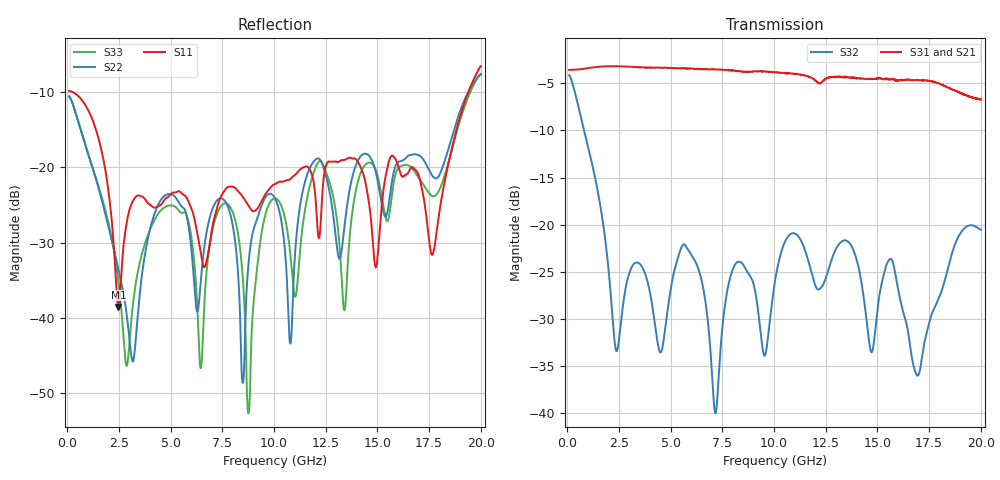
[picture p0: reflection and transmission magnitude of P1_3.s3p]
!The following data was pulled from an Agilent PNA
!This sNp file was generated from the data in the RF Test software
!NOTE:  Smoothing/Math/Corrections applied on any given trace ARE included in the data saved here
# MHz S dB R 50
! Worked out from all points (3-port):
!   6401 points, 100 MHz to 20 GHz, reference 50 ohm
!   strongest paths, dB at 100 MHz, 5.075 GHz, 10.05 GHz, 15.03 GHz, 20 GHz:
!     S31: -3.6, -3.4, -3.8, -4.5, -6.7
!     S21: -3.6, -3.4, -3.9, -4.6, -6.9
!     S32: -4.1, -26.0, -26.0, -28.6, -20.5
!   lowest |S11| = -38.5 dB at 2.485 GHz (marker M1), VSWR 1.02, Z = 49.9 + j1.17 ohm
!   |S11| at or under -10 dB: 236.6 MHz to 19.4 GHz (19.16 GHz wide, 195 % of centre)
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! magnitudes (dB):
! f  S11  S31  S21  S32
! 100 MHz  -9.9  -3.6  -3.6  -4.1
! 2.485 GHz  -38.5  -3.2  -3.2  -32.6
! 6.462 GHz  -31.3  -3.5  -3.5  -25.5
! 7.789 GHz  -22.6  -3.6  -3.6  -26.5
! 8.769 GHz  -25.1  -3.8  -3.8  -25.2
! 10.05 GHz  -22.2  -3.8  -3.9  -26.0
! 10.79 GHz  -21.6  -3.9  -4.0  -21.0
! 11.96 GHz  -22.7  -4.6  -4.6  -26.2
! 17.66 GHz  -31.6  -4.8  -5.0  -29.2
! 20 GHz  -6.6  -6.7  -6.9  -20.5
